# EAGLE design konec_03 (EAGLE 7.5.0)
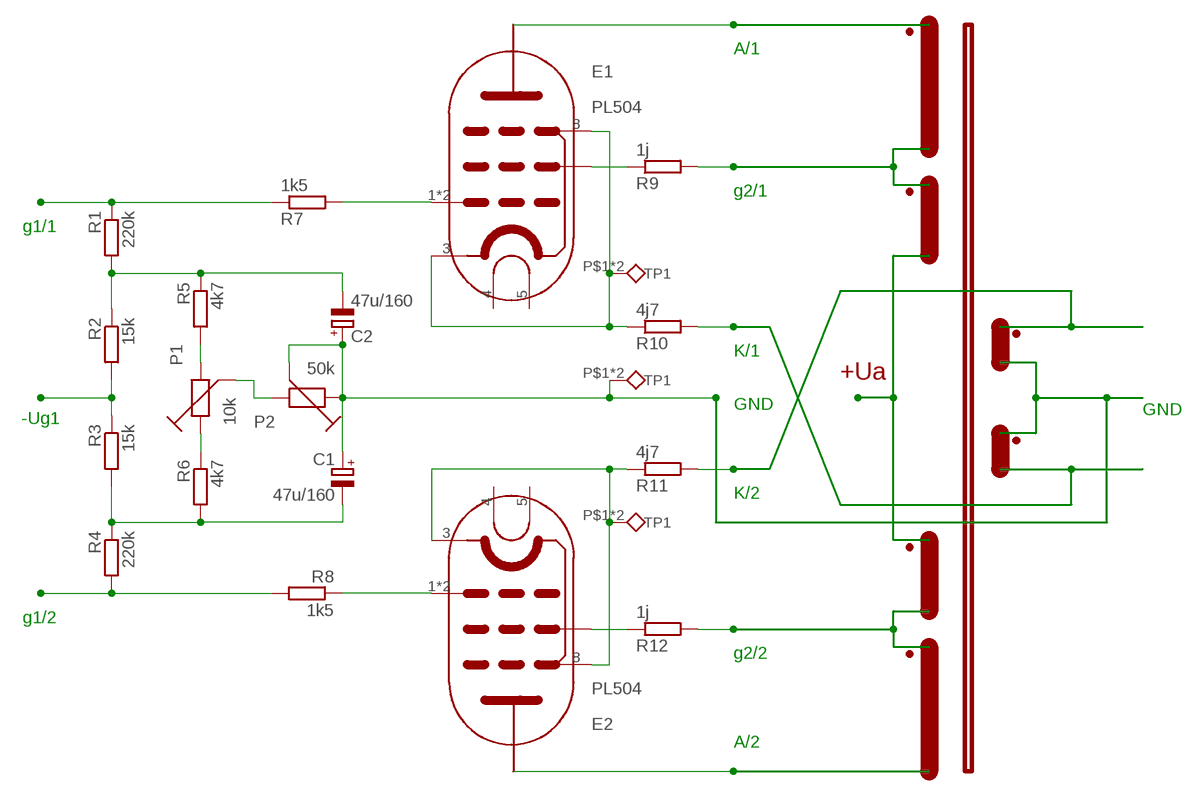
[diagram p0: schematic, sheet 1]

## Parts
C1  47u/160  CPOL-EUE2.5-7  [E2,5-7]
C2  47u/160  CPOL-EUE2.5-7  [E2,5-7]
E1  PL504  PL504HALF  [MAGNOVAL-HALF]
E2  PL504  PL504HALF  [MAGNOVAL-HALF]
P1  10k  P15VHALF  [P15V-HALF]
P2  50k  P15VHALF  [P15V-HALF]
R1  220k  R-EU_0207/10-HALF  [0207/10-HALF]
R2  15k  R-EU_0207/10-HALF  [0207/10-HALF]
R3  15k  R-EU_0207/10-HALF  [0207/10-HALF]
R4  220k  R-EU_0207/10-HALF  [0207/10-HALF]
R5  4k7  R-EU_0207/10-HALF  [0207/10-HALF]
R6  4k7  R-EU_0207/10-HALF  [0207/10-HALF]
R7  1k5  R-EU_0207/10-HALF  [0207/10-HALF]
R8  1k5  R-EU_0207/10-HALF  [0207/10-HALF]
R9  1j  R-EU_0207/10-HALF  [0207/10-HALF]
R10  4j7  R-EU_0207/10-HALF  [0207/10-HALF]
R11  4j7  R-EU_0207/10-HALF  [0207/10-HALF]
R12  1j  R-EU_0207/10-HALF  [0207/10-HALF]
U$3  TESTPINHALF  [TESTPIN2-HALF]
U$5  TESTPINHALF  [TESTPIN2-HALF]
U$7  TESTPINHALF  [TESTPIN2-HALF]

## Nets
-UG1: R2.2 R3.1
GND: C1.+ C2.+ P2.P$1 P2.P$3 U$7.P$1(TP1) U$7.P$2(TP1)
IN1: R4.2 R8.2
IN2: R1.1 R7.1
N$1: E2.1(G1) E2.2(G1) R8.1
N$3: E1.1(G1) E1.2(G1) R7.2
N$4: P1.P$3 R6.1
N$5: P1.P$1 P2.P$2
N$6: P1.P$2 R5.2
N$10: E2.6(G2) E2.7(G2) R12.1
N$11: E2.3(K) E2.8(G3) R11.1 U$5.P$1(TP1) U$5.P$2(TP1)
N$12: E1.3(K) E1.8(G3) R10.1 U$3.P$1(TP1) U$3.P$2(TP1)
N$13: E1.6(G2) E1.7(G2) R9.1
N$23: C1.- R3.2 R4.1 R6.2
N$24: C2.- R1.2 R2.1 R5.1
UG2-1: R12.2
UG2-2: R9.2
UK-1: R11.2
UK-2: R10.2
Unconnected: E1.4(F1) E1.5(F2) E2.4(F1) E2.5(F2)

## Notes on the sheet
- A/1
- g2/1
- g1/1
- K/1
- +Ua
- GND
- -Ug1 | GND
- K/2
- g1/2
- g2/2
- A/2

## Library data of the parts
C1 C2 = rcl:CPOL-EU: POLARIZED CAPACITOR, European symbol
E1 E2 = PL500:PL504
P1 P2 = lampy04:P15V
R1-R12 = rcl:R-EU_: RESISTOR, European symbol
U$3 U$5 U$7 = lampy04:TESTPIN

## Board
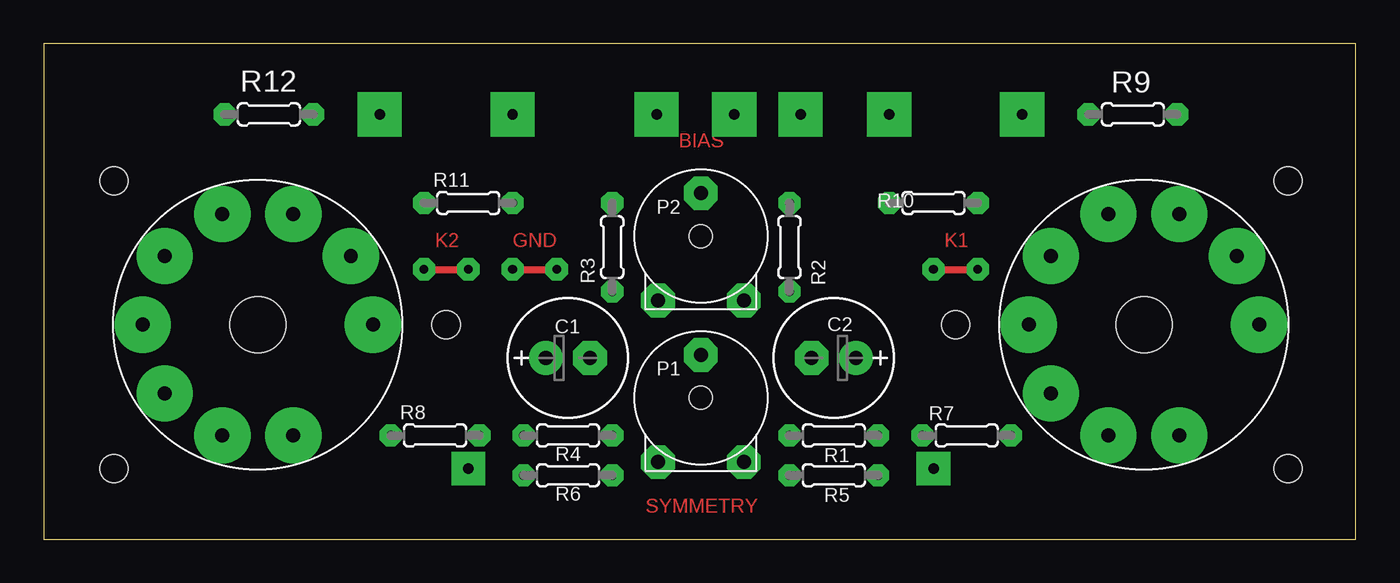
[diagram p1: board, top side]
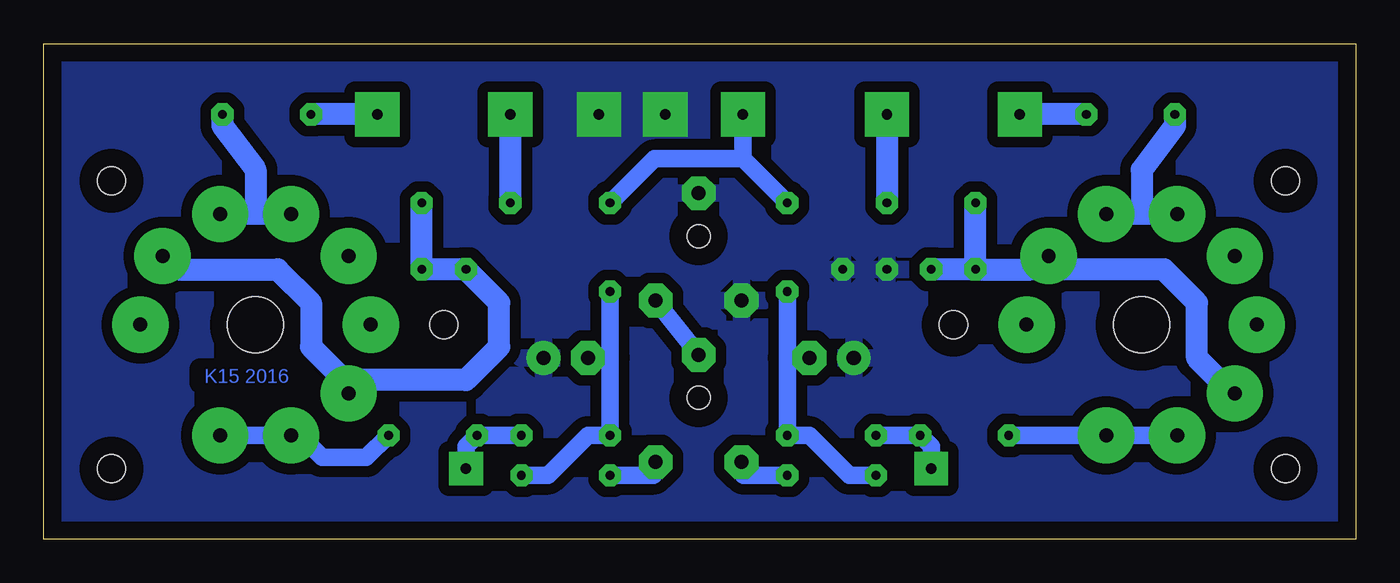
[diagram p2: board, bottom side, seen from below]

Size 75.23 x 28.43 mm. Coordinates in mm from the lower left corner, seen from the top.
Outline: 0,28.43 0,0 75.23,0 75.23,28.43 0,28.43
Copper layers (1*16): Top 0.035mm / dielectric 1.5mm / Bottom 0.035mm
Design rules "default": minimum track width 10mil, minimum drill 24mil, track to track 8mil, track to pad 8mil, pad to pad 8mil, via to via 8mil, smd to smd 8mil, copper to edge 40mil, drill to drill 8mil, minimum pad ring 10mil, minimum via ring 8mil, stop-mask expansion 4mil, vias tented up to drill 0mil, thermal gap 10mil
Holes 1.6 mm at 4.03,20.56 4.03,4.05 23.08,12.3 52.29,12.3 71.34,20.56 71.34,4.05
Holes 3.2 mm at 12.28,12.3 63.08,12.3

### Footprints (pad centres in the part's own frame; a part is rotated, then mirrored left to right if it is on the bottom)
E2,5-7 = drill 0.813 pad 1.93: + -1.27,0 | drill 0.813 pad 1.93 octagon: - 1.27,0
MAGNOVAL-HALF = drill 0.8 pad 3.226: 1 2.032,-6.35; 2 -2.032,-6.35; 3 -5.334,-3.937; 4 -6.604,0; 5 -5.334,3.937; 6 -2.032,6.35; 7 2.032,6.35; 8 5.334,3.937; 9 6.604,0
P15V-HALF = drill 0.8 pad 1.93 octagon: P$1 0,2.46; P$2 2.46,-3.69; P$3 -2.46,-3.69 | hole 1.3: 0,0
0207/10-HALF = drill 0.5 pad 1.27 octagon: 1 -2.54,0; 2 2.54,0
TESTPIN2-HALF = drill 0.5 pad 1.27 octagon: P$1 -1.27,0; P$2 1.27,0

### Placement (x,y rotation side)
C1  30.06,10.4 0 top
C2  45.3,10.4 180 top
E1  63.08,12.3 0 top
E2  12.28,12.3 0 top
P1  37.68,8.11 0 top
P2  37.68,17.38 0 top
R1  45.3,5.95 180 top
R2  42.76,16.75 90 top
R3  32.6,16.75 270 top
R4  30.06,5.95 180 top
R5  45.3,3.67 180 top
R6  30.06,3.67 180 top
R7  52.92,5.95 0 top
R8  22.44,5.95 0 top
R9  62.45,24.37 180 top
R10  51.02,19.29 180 top
R11  24.35,19.29 0 top
R12  12.92,24.37 0 top
U$3  52.29,15.48 180 top
U$5  23.08,15.48 0 top
U$7  28.16,15.48 0 top

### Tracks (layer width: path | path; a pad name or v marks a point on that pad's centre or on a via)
-UG1  (via drill 0.6 pad 2.54)
  Bottom 1.016: 35.14,21.83 40.22,21.83 R2.2 | R3.1 35.14,21.83 | v35.14,24.37 35.14,21.83
GND  (via drill 0.5, 0.6 pad 2.54)
  Top 0.406: U$7.P$1 U$7.P$2
  other vias: 39.59,24.37 28.79,10.4 46.57,10.4 43.4,24.37
  pour Bottom (isolate 0.61): 74.89,28.18 74.89,-0.02 0.34,-0.02 0.34,28.18
IN1  (via drill 0.6 pad 1.93)
  Bottom 1.016: R4.2 R8.2 24.35,5.32 v24.35,4.05
IN2  (via drill 0.6 pad 1.93)
  Bottom 1.016: R1.1 R7.1 51.02,5.32 v51.02,4.05
N$1
  Bottom 1.016: E2.2 E2.1 R8.1
N$3
  Bottom 0.61: E1.2 60.54,5.95
  Bottom 1.016: E1.1 E1.2 | 60.54,5.95 59.27,4.68 56.73,4.68 R7.2
N$4
  Bottom 1.016: R6.1 35.1,3.67 P1.P$3
N$5
  Bottom 0.813: P1.P$1 37.68,10.6
  Bottom 1.016: 37.68,10.6 P2.P$2
N$6
  Bottom 1.016: R5.2 40.26,3.67 P1.P$2
N$7  (via drill 0.5)
  other vias: 31.33,10.4
N$8  (via drill 0.5)
  other vias: 44.03,10.4
N$10
  Bottom 1.27: E2.6 12.28,18.65 | 12.28,18.65 E2.7 | R12.1 10.38,23.73 12.28,21.19 12.28,18.65
N$11
  Top 0.406: U$5.P$1 U$5.P$2
  Bottom 1.27: U$5.P$1 18.63,15.48 18.25,15.73 18.22,15.76 | E2.8 18.22,15.76 | U$5.P$1 R11.1 | U$5.P$1 U$5.P$2 | E2.3 7.07,8.37 9.11,10.4 9.11,13.57 11.01,15.48 17.94,15.48 18.22,15.76
N$12
  Top 0.406: U$3.P$2 U$3.P$1
  Bottom 1.27: E1.3 57.75,8.88 | 57.75,8.88 57.37,9.13 51.02,9.13 49.11,11.03 49.11,13.57 U$3.P$2 U$3.P$1 R10.1 | E1.8 68.29,16.24 67.53,15.48 61.81,15.48 59.91,13.57 59.91,11.03 57.75,8.88
N$13
  Bottom 1.27: E1.6 63.08,18.65 | 63.08,18.65 E1.7 65.11,18.78 | R9.1 64.99,23.73 63.08,21.19 63.08,18.65
N$23
  Bottom 1.016: R3.2 32.6,10.4 | 32.6,10.4 R4.1 31.33,5.95 29.05,3.67 R6.2 | C1.- 32.6,10.4
N$24
  Bottom 0.813: C2.- 42.76,10.4
  Bottom 1.016: R2.1 42.76,10.4 R1.2 44.03,5.95 46.32,3.67 R5.1
UG2-1  (via drill 0.6 pad 2.54)
  Bottom 1.27: R12.2 v19.27,24.37
UG2-2  (via drill 0.6 pad 2.54)
  Bottom 1.27: v56.1,24.37 R9.2
UK-1  (via drill 0.6 pad 2.54)
  Bottom 1.27: v26.89,24.37 R11.2
UK-2  (via drill 0.6 pad 2.54)
  Bottom 1.27: R10.2 v48.48,24.37

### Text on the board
Top: BIAS | K2 | GND | K1 | SYMMETRY
Bottom: K15 2016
